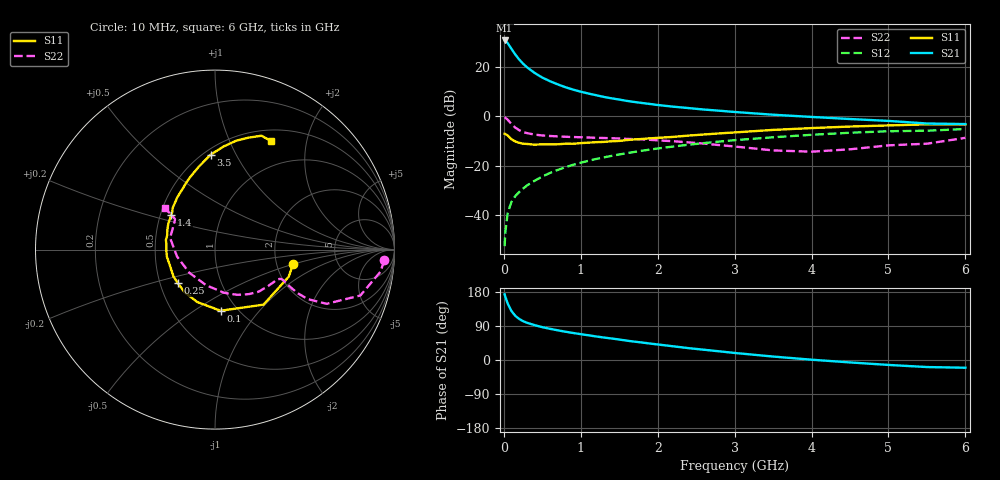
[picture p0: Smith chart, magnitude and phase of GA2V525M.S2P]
! Infineon Technologies  Discrete & RF Semiconductors
! BF775
! Si NPN RF Bipolar Junction Transistor in SOT23
! VCE = 2.5 V  IC = 25 mA
! Common Emitter S-Parameters:  May  1996
# GHz  S  MA  R  50
!  f  S11  S21  S12  S22
! GHz  MAG  ANG  MAG  ANG  MAG  ANG  MAG  ANG
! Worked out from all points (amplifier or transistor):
!   36 points, 10 MHz to 6 GHz, reference 50 ohm
!   highest |S21| = 30.5 dB at 10 MHz (marker M1)
!   |S21| within 3 dB of that: start of sweep to 91 MHz
!   unconditionally stable (mu >= 1): 281.8 MHz to 3.595 GHz; 5.45 GHz to 5.663 GHz
!   at 250 MHz: K = 0.97, MSG = 25.2 dB, |S12| = -29.2 dB
!   at 1.4 GHz: K = 1.16, MAG = 9.2 dB, |S12| = -16.0 dB
!   at 6 GHz: K = 0.99, MSG = 1.0 dB, |S12| = -5.2 dB
!   S11 on the Smith chart (normalised r, x): 10 MHz: 2.47, -0.50; 100 MHz: 0.84, -0.65; 250 MHz: 0.62, -0.25; 1.4 GHz: 0.57, +0.24; 3.5 GHz: 0.54, +0.79; 6 GHz: 0.64, +1.44
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0.01  0.4424 -10.6  33.59 173.2  0.0024 84.2  0.9456 -3.6
0.02  0.4376 -20.2  32.95 166.6  0.0047 82.4  0.9292 -7.7
0.05  0.4088 -48.6  29.74 149.2  0.0112 73.9  0.8493 -17.5
0.1  0.342 -84.8  22.64 129.0  0.0189 67.0  0.6916 -25.9
0.15  0.3084 -108.9  17.4 116.3  0.0246 66.2  0.5859 -28.1
0.2  0.2911 -126.0  13.87 108.3  0.0297 66.3  0.5216 -27.8
0.25  0.2787 -138.2  11.41 102.5  0.0347 68.0  0.4805 -26.8
0.3  0.2758 -146.9  9.713 98.3  0.0401 68.9  0.4561 -26.0
0.4  0.2666 -161.3  7.447 92.0  0.05 70.5  0.4255 -24.6
0.5  0.271 -171.7  5.997 86.7  0.0608 71.4  0.4087 -23.9
0.6  0.2709 -178.5  5.064 82.3  0.0718 71.3  0.3986 -24.1
0.7  0.2717 174.6  4.38 78.3  0.0824 71.3  0.3917 -24.8
0.8  0.2788 168.9  3.842 74.7  0.0937 70.7  0.3848 -25.6
0.9  0.2782 163.2  3.429 71.3  0.1046 69.8  0.38 -26.7
1.1  0.2928 153.9  2.858 65.2  0.1261 68.7  0.3718 -29.7
1.4  0.3119 141.9  2.291 56.8  0.1585 65.6  0.3593 -34.6
1.7  0.3399 131.9  1.93 48.4  0.1907 62.4  0.3439 -40.4
2.2  0.3824 118.4  1.555 36.2  0.2445 56.4  0.3129 -52.3
3.5  0.529 92.7  1.07 9.1  0.376 39.0  0.2042 -104.2
4.5  0.6187 78.9  0.877 -6.4  0.4637 24.7  0.2149 -169.6
5.5  0.6853 67.8  0.712 -18.6  0.5094 9.4  0.279 142.6
6  0.681 62.9  0.693 -20.4  0.5512 5.2  0.3662 140.2
